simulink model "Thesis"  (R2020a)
settings: Solver=ode15s  StartTime=0.0  StopTime=1440  MaxStep=1  RelTol=1e-3
model workspace (MAT data in the model file):
  SDO_OutputTimes = [0 45 72 95 129 186 320 430 960 1290]
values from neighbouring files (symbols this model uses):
  BR = 5000    [VariablesHighBFloretsSR.m]    (also in VariablesHighBPowderSR.m; VariablesLowBFloretsSR.m; VariablesMedBFloretsSR.m; VariablesNoBFloretsSR.m)
  Cgl0 = 621.875    [VariablesHighBFloretsSR.m]    (also in VariablesHighBPowderSR.m = 383.33; VariablesLowBFloretsSR.m = 708.333; VariablesMedBFloretsSR.m = 667.70833; VariablesNoBFloretsSR.m = 734.375)
  ITC0 = 115.625    [VariablesHighBFloretsSR.m]    (also in VariablesHighBPowderSR.m = 354.17; VariablesLowBFloretsSR.m = 2.65154545455; VariablesMedBFloretsSR.m = 2.40689655172; VariablesNoBFloretsSR.m = 3.125)
  ka = 0.17952    [VariablesHighBFloretsSR.m]    (also in VariablesHighBPowderSR.m; VariablesLowBFloretsSR.m; VariablesMedBFloretsSR.m; VariablesNoBFloretsSR.m)
  ke = 0.024    [VariablesHighBFloretsSR.m]    (also in VariablesHighBPowderSR.m; VariablesLowBFloretsSR.m; VariablesMedBFloretsSR.m; VariablesNoBFloretsSR.m)
  keni = 0.0015    [VariablesHighBFloretsSR.m]    (also in VariablesHighBPowderSR.m; VariablesLowBFloretsSR.m; VariablesMedBFloretsSR.m; VariablesNoBFloretsSR.m)
  kf = 0.00333    [VariablesHighBFloretsSR.m]    (also in VariablesHighBPowderSR.m; VariablesLowBFloretsSR.m; VariablesMedBFloretsSR.m; VariablesNoBFloretsSR.m)
  Ki = 893.018606646    [VariablesHighBFloretsSR.m]    (also in VariablesHighBPowderSR.m; VariablesLowBFloretsSR.m; VariablesMedBFloretsSR.m; VariablesNoBFloretsSR.m)
  Km = 110.161136443    [VariablesHighBFloretsSR.m]    (also in VariablesHighBPowderSR.m; VariablesLowBFloretsSR.m; VariablesMedBFloretsSR.m; VariablesNoBFloretsSR.m)
  ktli = 0.002682    [VariablesHighBFloretsSR.m]    (also in VariablesHighBPowderSR.m; VariablesLowBFloretsSR.m; VariablesMedBFloretsSR.m; VariablesNoBFloretsSR.m)
  ktsi = 0.03518    [VariablesHighBFloretsSR.m]    (also in VariablesHighBPowderSR.m; VariablesLowBFloretsSR.m; VariablesMedBFloretsSR.m; VariablesNoBFloretsSR.m = 0.0351)
  M = 30    [VariablesHighBFloretsSR.m]    (also in VariablesHighBPowderSR.m; VariablesLowBFloretsSR.m; VariablesMedBFloretsSR.m; VariablesNoBFloretsSR.m)
  MYR = 0.0348960299    [VariablesHighBFloretsSR.m]    (also in VariablesHighBPowderSR.m; VariablesLowBFloretsSR.m = 0.000562839; VariablesMedBFloretsSR.m = 0.006528935; VariablesNoBFloretsSR.m = 1.12568e-05)
  NLI = 7    [VariablesHighBFloretsSR.m]    (also in VariablesHighBPowderSR.m; VariablesLowBFloretsSR.m; VariablesMedBFloretsSR.m; VariablesNoBFloretsSR.m)
  NSI = 6    [VariablesHighBFloretsSR.m]    (also in VariablesHighBPowderSR.m; VariablesLowBFloretsSR.m; VariablesMedBFloretsSR.m; VariablesNoBFloretsSR.m)
  SH = 0.02    [VariablesHighBFloretsSR.m]    (also in VariablesHighBPowderSR.m; VariablesLowBFloretsSR.m; VariablesMedBFloretsSR.m; VariablesNoBFloretsSR.m)
  SRR = 0.4737    [VariablesHighBFloretsSR.m]    (also in VariablesHighBPowderSR.m; VariablesLowBFloretsSR.m; VariablesMedBFloretsSR.m; VariablesNoBFloretsSR.m)
  St = 30    [VariablesHighBFloretsSR.m]    (also in VariablesHighBPowderSR.m; VariablesLowBFloretsSR.m; VariablesMedBFloretsSR.m; VariablesNoBFloretsSR.m)
  V1 = 0.096    [VariablesHighBFloretsSR.m]    (also in VariablesHighBPowderSR.m; VariablesLowBFloretsSR.m; VariablesMedBFloretsSR.m; VariablesNoBFloretsSR.m)
  V18 = 5    [VariablesHighBFloretsSR.m]    (also in VariablesHighBPowderSR.m; VariablesLowBFloretsSR.m; VariablesMedBFloretsSR.m; VariablesNoBFloretsSR.m)
  V2 = 0.05    [VariablesHighBFloretsSR.m]    (also in VariablesHighBPowderSR.m; VariablesLowBFloretsSR.m; VariablesMedBFloretsSR.m; VariablesNoBFloretsSR.m)
  V3 = 0.15    [VariablesHighBFloretsSR.m]    (also in VariablesHighBPowderSR.m; VariablesLowBFloretsSR.m; VariablesMedBFloretsSR.m; VariablesNoBFloretsSR.m)
  V4 = 0.2    [VariablesHighBFloretsSR.m]    (also in VariablesHighBPowderSR.m; VariablesLowBFloretsSR.m; VariablesMedBFloretsSR.m; VariablesNoBFloretsSR.m)
  VLI = 3.4    [VariablesHighBFloretsSR.m]    (also in VariablesHighBPowderSR.m; VariablesLowBFloretsSR.m; VariablesMedBFloretsSR.m; VariablesNoBFloretsSR.m)
  Vmax = 2070    [VariablesHighBFloretsSR.m]    (also in VariablesHighBPowderSR.m; VariablesLowBFloretsSR.m; VariablesMedBFloretsSR.m; VariablesNoBFloretsSR.m)
  VSI = 1.5    [VariablesHighBFloretsSR.m]    (also in VariablesHighBPowderSR.m; VariablesLowBFloretsSR.m; VariablesMedBFloretsSR.m; VariablesNoBFloretsSR.m)
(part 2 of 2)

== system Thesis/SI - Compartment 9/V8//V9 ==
  Divide : Product  Inputs=*/
  SI # compartments : Constant  Value=NSI
  SI # compartments1 : Constant  Value=NSI
  SI Volume : Constant  Value=VSI
  SI Volume1 : Constant  Value=VSI
  "V8=VSI/NSI, SI 1" : Product  Inputs=*/
  "V9=VSI/NSI, SI " : Product  Inputs=*/
  Out1 : Outport
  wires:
  Divide/1 -> Out1/1
  SI Volume/1 -> "V9=VSI/NSI, SI "/1
  SI # compartments/1 -> "V9=VSI/NSI, SI "/2
  "V9=VSI/NSI, SI "/1 -> Divide/2  "V9"
  "V8=VSI/NSI, SI 1"/1 -> Divide/1  "V8"
  SI # compartments1/1 -> "V8=VSI/NSI, SI 1"/2
  SI Volume1/1 -> "V8=VSI/NSI, SI 1"/1

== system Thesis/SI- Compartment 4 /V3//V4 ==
  Divide : Product  Inputs=*/
  V3 : Constant  Value=V3
  V4 : Constant  Value=V4
  Out1 : Outport
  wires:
  V3/1 -> Divide/1
  V4/1 -> Divide/2
  Divide/1 -> Out1/1
